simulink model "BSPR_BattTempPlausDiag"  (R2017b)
settings: Solver=FixedStepDiscrete  StartTime=0.0  StopTime=10.0  FixedStep=0.02  RelTol=1e-3  EnableMultiTasking=on
undefined symbols (not defined in the file): bin2dec, BSPR_cntBattTCnstErrDet_C, BSPR_cntBattTCnstErrHeal_C, BSPR_cntBattTHopErrDet_C, BSPR_cntBattTHopErrHeal_C, BSPR_cntBattTPlausDiag_CW, BSPR_cntCellTPlausDiag_CW, BSPR_cofBattTLowPassK_C, BSPR_tBattTCnstFaultThres_C, BSPR_tBattTempCnstHi_C, BSPR_tBattTempCnstLo_C, BSPR_tBattTempCnstThres_C, BSPR_tBattTempEnvtDiff_C, BSPR_tBattTHopFaultThres_C, BSPR_tBusbarTCnstFaultThres_C, BSPR_tBusbarTCnstHealThres_C, BSPR_tCellTCnstFaultThres_C, BSPR_tCellTCnstHealThres_C, BSPR_tiBattTCnstErrDet_C, BSPR_tiBattTCnstErrHeal_C
libraries: simulink x12
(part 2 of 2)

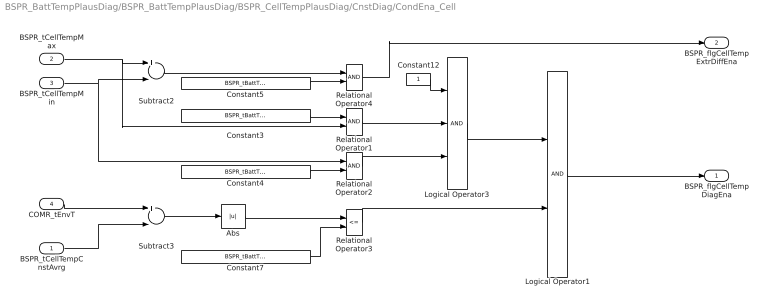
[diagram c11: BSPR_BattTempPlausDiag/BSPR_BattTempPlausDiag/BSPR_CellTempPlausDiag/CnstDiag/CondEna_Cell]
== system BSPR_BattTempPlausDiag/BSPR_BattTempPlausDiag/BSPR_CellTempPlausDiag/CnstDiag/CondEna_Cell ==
  BSPR_tCellTempCnstAvrg : Inport
  BSPR_tCellTempMax : Inport  Port=2
  BSPR_tCellTempMin : Inport  Port=3
  COMR_tEnvT : Inport  Port=4
  Abs : Abs
  Constant12 : Constant  OutDataTypeStr=boolean
  Constant3 : Constant  Value=BSPR_tBattTempCnstHi_C
  Constant4 : Constant  Value=BSPR_tBattTempCnstLo_C
  Constant5 : Constant  Value=BSPR_tBattTempCnstThres_C
  Constant7 : Constant  Value=BSPR_tBattTempEnvtDiff_C
  Logical Operator1 : Logic  AllPortsSameDT=off  OutDataTypeStr=boolean
  Logical Operator3 : Logic  Inputs=3  AllPortsSameDT=off  OutDataTypeStr=boolean
  Relational Operator1 : RelationalOperator  OutDataTypeStr=boolean  RndMeth=Simplest
  Relational Operator2 : RelationalOperator  OutDataTypeStr=boolean  RndMeth=Simplest
  Relational Operator3 : RelationalOperator  Operator=<=  OutDataTypeStr=boolean  RndMeth=Simplest
  Relational Operator4 : RelationalOperator  OutDataTypeStr=boolean  RndMeth=Simplest
  Subtract2 : Sum  Inputs=+-  OutDataTypeStr=uint8
  Subtract3 : Sum  Inputs=+-  OutDataTypeStr=single
  BSPR_flgCellTempDiagEna : Outport
  BSPR_flgCellTempExtrDiffEna : Outport  Port=2
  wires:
  Relational Operator4/1 -> BSPR_flgCellTempExtrDiffEna/1
  Relational Operator1/1 -> Logical Operator3/2
  Abs/1 -> Relational Operator3/1
  Logical Operator1/1 -> BSPR_flgCellTempDiagEna/1
  Relational Operator3/1 -> Logical Operator1/2
  Logical Operator3/1 -> Logical Operator1/1
  Constant7/1 -> Relational Operator3/2
  Subtract3/1 -> Abs/1
  BSPR_tCellTempCnstAvrg/1 -> Subtract3/2
  COMR_tEnvT/1 -> Subtract3/1
  Relational Operator2/1 -> Logical Operator3/3
  Constant4/1 -> Relational Operator2/2
  Constant3/1 -> Relational Operator1/1
  Subtract2/1 -> Relational Operator4/1
  Constant5/1 -> Relational Operator4/2
  BSPR_tCellTempMin/1 -> Subtract2/2, Relational Operator2/1
  BSPR_tCellTempMax/1 -> Subtract2/1, Relational Operator1/2
  Constant12/1 -> Logical Operator3/1

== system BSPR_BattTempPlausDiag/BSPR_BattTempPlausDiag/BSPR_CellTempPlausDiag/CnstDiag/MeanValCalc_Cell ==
  BSPR_cntCellTSnsrNum : Inport
  BSPR_tCellTemp_A : Inport  Port=2
  BSPR_tCellTempCnstAvrg : Inport  Port=3
  MeanValCalc_Cell : Stateflow chart  TreatAsAtomicUnit=on
  BSPR_tAvrgCellTempFlt : Outport
  BSPR_tSumCellTempVari : Outport  Port=2
  BSPR_tSumCellTempFlt : Outport  Port=3
  BSPR_tCellTempVari_A : Outport  Port=4
  BSPR_tAvrgCellTempVari : Outport  Port=5
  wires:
  BSPR_tCellTempCnstAvrg/1 -> MeanValCalc_Cell/2(BSPR_tBattTempCnstAvrg)
  BSPR_tCellTemp_A/1 -> MeanValCalc_Cell/1(BSPR_tBattTemp_A)
  MeanValCalc_Cell/4(BSPR_tBattTempVari_A) -> BSPR_tCellTempVari_A/1
  MeanValCalc_Cell/1(BSPR_tAvrgBattTempFlt) -> BSPR_tAvrgCellTempFlt/1
  MeanValCalc_Cell/2(BSPR_tSumBattTempVari) -> BSPR_tSumCellTempVari/1
  MeanValCalc_Cell/5(BSPR_tAvrgBattTempVari) -> BSPR_tAvrgCellTempVari/1
  MeanValCalc_Cell/3(BSPR_tSumBattTempFlt) -> BSPR_tSumCellTempFlt/1
  BSPR_cntCellTSnsrNum/1 -> MeanValCalc_Cell/3(BSPR_cntBattTSnsrNum)

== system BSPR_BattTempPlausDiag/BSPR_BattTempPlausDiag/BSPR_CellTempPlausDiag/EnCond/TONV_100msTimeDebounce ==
  note: Turn On Delay Time Deboune
  u : Inport
  T : Inport  Port=2
  Add : Sum
  Constant1 : Constant  Value=0  OutDataTypeStr=single
  Constant2 : Constant  OutDataTypeStr=uint8
  Constant3 : Constant  Value=0  OutDataTypeStr=uint8
  Constant4 : Constant  Value=0.1  OutDataTypeStr=single
  Delay : Delay  DelayLength=1  InitialCondition=0
  MinMax : MinMax  Inputs=2
  Product : Product  OutMin=[0]  OutMax=[65535]  OutDataTypeStr=single
  Relational Operator : RelationalOperator  Operator=>  OutDataTypeStr=boolean  RndMeth=Simplest
  Switch : Switch  Criteria=u2 ~= 0
  Switch1 : Switch  Criteria=u2 ~= 0
  y : Outport
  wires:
  MinMax/1 -> Add/2
  T/1 -> Relational Operator/2, MinMax/1
  Relational Operator/1 -> y/1
  Delay/1 -> MinMax/2
  Switch/1 -> Add/1
  Product/1 -> Delay/1, Relational Operator/1
  Add/1 -> Product/2
  Constant1/1 -> Switch/3
  Constant4/1 -> Switch/1
  u/1 -> Switch/2, Switch1/2
  Constant2/1 -> Switch1/1
  Constant3/1 -> Switch1/3
  Switch1/1 -> Product/1

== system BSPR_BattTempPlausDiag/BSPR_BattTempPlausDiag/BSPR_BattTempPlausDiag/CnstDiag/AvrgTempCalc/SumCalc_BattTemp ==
  BSPR_tBattTemp_A : Inport
  BSPR_cntBattTSnsrNum : Inport  Port=2
  SumCalc_BattTemp : Stateflow chart  TreatAsAtomicUnit=on
  BSPR_tSumBattTemp : Outport
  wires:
  BSPR_cntBattTSnsrNum/1 -> SumCalc_BattTemp/2(BSPR_cntBattTSnsrNum)
  BSPR_tBattTemp_A/1 -> SumCalc_BattTemp/1(BSPR_tBattTemp_A)
  SumCalc_BattTemp/1(BSPR_uSumBattTemp) -> BSPR_tSumBattTemp/1

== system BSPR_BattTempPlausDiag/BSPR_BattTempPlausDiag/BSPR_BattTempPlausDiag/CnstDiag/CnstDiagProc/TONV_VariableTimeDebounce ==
  note: Turn On Delay Time Deboune
  u : Inport
  T : Inport  Port=2
  dT : Inport  Port=3
  Add : Sum
  Constant1 : Constant  Value=0  OutDataTypeStr=single
  Constant2 : Constant  OutDataTypeStr=uint8
  Constant3 : Constant  Value=0  OutDataTypeStr=uint8
  Delay : Delay  DelayLength=1  InitialCondition=0
  MinMax : MinMax  Inputs=2
  Product : Product  OutMin=[0]  OutMax=[65535]  OutDataTypeStr=single
  Relational Operator : RelationalOperator  Operator=>  OutDataTypeStr=boolean  RndMeth=Simplest
  Switch : Switch  Criteria=u2 ~= 0
  Switch1 : Switch  Criteria=u2 ~= 0
  y : Outport
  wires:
  Switch1/1 -> Product/1
  Constant3/1 -> Switch1/3
  Constant2/1 -> Switch1/1
  u/1 -> Switch1/2, Switch/2
  dT/1 -> Switch/1
  Constant1/1 -> Switch/3
  Add/1 -> Product/2
  Product/1 -> Relational Operator/1, Delay/1
  Switch/1 -> Add/1
  Delay/1 -> MinMax/2
  Relational Operator/1 -> y/1
  T/1 -> MinMax/1, Relational Operator/2
  MinMax/1 -> Add/2

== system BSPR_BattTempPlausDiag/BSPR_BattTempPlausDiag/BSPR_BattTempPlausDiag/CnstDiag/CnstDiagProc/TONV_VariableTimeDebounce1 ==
  note: Turn On Delay Time Deboune
  u : Inport
  T : Inport  Port=2
  dT : Inport  Port=3
  Add : Sum
  Constant1 : Constant  Value=0  OutDataTypeStr=single
  Constant2 : Constant  OutDataTypeStr=uint8
  Constant3 : Constant  Value=0  OutDataTypeStr=uint8
  Delay : Delay  DelayLength=1  InitialCondition=0
  MinMax : MinMax  Inputs=2
  Product : Product  OutMin=[0]  OutMax=[65535]  OutDataTypeStr=single
  Relational Operator : RelationalOperator  Operator=>  OutDataTypeStr=boolean  RndMeth=Simplest
  Switch : Switch  Criteria=u2 ~= 0
  Switch1 : Switch  Criteria=u2 ~= 0
  y : Outport
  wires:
  MinMax/1 -> Add/2
  T/1 -> Relational Operator/2, MinMax/1
  Relational Operator/1 -> y/1
  Delay/1 -> MinMax/2
  Switch/1 -> Add/1
  Product/1 -> Delay/1, Relational Operator/1
  Add/1 -> Product/2
  Constant1/1 -> Switch/3
  dT/1 -> Switch/1
  u/1 -> Switch/2, Switch1/2
  Constant2/1 -> Switch1/1
  Constant3/1 -> Switch1/3
  Switch1/1 -> Product/1

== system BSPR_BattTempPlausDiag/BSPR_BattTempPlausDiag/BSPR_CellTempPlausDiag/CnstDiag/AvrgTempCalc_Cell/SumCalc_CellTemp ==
  BSPR_tCellTemp_A : Inport
  BSPR_cntCellTSnsrNum : Inport  Port=2
  SumCalc_CellTemp : Stateflow chart  TreatAsAtomicUnit=on
  BSPR_tSumCellTemp : Outport
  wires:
  SumCalc_CellTemp/1(BSPR_uSumBattTemp) -> BSPR_tSumCellTemp/1
  BSPR_tCellTemp_A/1 -> SumCalc_CellTemp/1(BSPR_tBattTemp_A)
  BSPR_cntCellTSnsrNum/1 -> SumCalc_CellTemp/2(BSPR_cntBattTSnsrNum)

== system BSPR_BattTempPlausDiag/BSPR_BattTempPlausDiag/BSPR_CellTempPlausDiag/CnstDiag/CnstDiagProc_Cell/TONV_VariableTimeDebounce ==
  note: Turn On Delay Time Deboune
  u : Inport
  T : Inport  Port=2
  dT : Inport  Port=3
  Add : Sum
  Constant1 : Constant  Value=0  OutDataTypeStr=single
  Constant2 : Constant  OutDataTypeStr=uint8
  Constant3 : Constant  Value=0  OutDataTypeStr=uint8
  Delay : Delay  DelayLength=1  InitialCondition=0
  MinMax : MinMax  Inputs=2
  Product : Product  OutMin=[0]  OutMax=[65535]  OutDataTypeStr=single
  Relational Operator : RelationalOperator  Operator=>  OutDataTypeStr=boolean  RndMeth=Simplest
  Switch : Switch  Criteria=u2 ~= 0
  Switch1 : Switch  Criteria=u2 ~= 0
  y : Outport
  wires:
  Switch1/1 -> Product/1
  Constant3/1 -> Switch1/3
  Constant2/1 -> Switch1/1
  u/1 -> Switch1/2, Switch/2
  dT/1 -> Switch/1
  Constant1/1 -> Switch/3
  Add/1 -> Product/2
  Product/1 -> Relational Operator/1, Delay/1
  Switch/1 -> Add/1
  Delay/1 -> MinMax/2
  Relational Operator/1 -> y/1
  T/1 -> MinMax/1, Relational Operator/2
  MinMax/1 -> Add/2

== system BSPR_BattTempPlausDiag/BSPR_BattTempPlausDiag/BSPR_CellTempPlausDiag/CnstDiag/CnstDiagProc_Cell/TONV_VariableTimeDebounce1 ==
  note: Turn On Delay Time Deboune
  u : Inport
  T : Inport  Port=2
  dT : Inport  Port=3
  Add : Sum
  Constant1 : Constant  Value=0  OutDataTypeStr=single
  Constant2 : Constant  OutDataTypeStr=uint8
  Constant3 : Constant  Value=0  OutDataTypeStr=uint8
  Delay : Delay  DelayLength=1  InitialCondition=0
  MinMax : MinMax  Inputs=2
  Product : Product  OutMin=[0]  OutMax=[65535]  OutDataTypeStr=single
  Relational Operator : RelationalOperator  Operator=>  OutDataTypeStr=boolean  RndMeth=Simplest
  Switch : Switch  Criteria=u2 ~= 0
  Switch1 : Switch  Criteria=u2 ~= 0
  y : Outport
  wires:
  MinMax/1 -> Add/2
  T/1 -> Relational Operator/2, MinMax/1
  Relational Operator/1 -> y/1
  Delay/1 -> MinMax/2
  Switch/1 -> Add/1
  Product/1 -> Delay/1, Relational Operator/1
  Add/1 -> Product/2
  Constant1/1 -> Switch/3
  dT/1 -> Switch/1
  u/1 -> Switch/2, Switch1/2
  Constant2/1 -> Switch1/1
  Constant3/1 -> Switch1/3
  Switch1/1 -> Product/1

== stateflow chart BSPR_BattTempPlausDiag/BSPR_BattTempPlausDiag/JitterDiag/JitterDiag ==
  state Ini_stt
    (default) -> (junction 142) : % ini
    (junction 138) -> (junction 143) : [i<BSPR_cntBattTSnsrNum]
    (junction 142) -> (junction 138) : {i=0;}
    (junction 143) -> (junction 139) : {BSPR_tBattTempDiag_A[i]=BSPR_tBattTemp_A[i]; BSPR_tBattTHopDiff_A[i]=0;}
    (junction 139) -> (junction 138) : {i = i + 1;}
    (junction 138) -> (junction 136)
  state DiagUCellProc_stt
    (default) -> (junction 10) : /*Compare */
    (junction 23) -> (junction 120) : [abs(BSPR_tBattTHopDiff_A[i])>=BSPR_tBattTHopFaultThres_C]
    (junction 9) -> (junction 23) : {[BSPR_tBattTempDiag_A[i],BSPR_tBattTHopDiff_A[i]]=LowPassK(BSPR_tBattTemp_A[i],BSPR_tBattTempDiag_A[i],BSPR_cofBattTLowPassK_C);}
    (junction 11) -> (junction 9) : [i<BSPR_cntBattTSnsrNum]
    (junction 10) -> (junction 11) : {i=0;}
    (junction 23) -> (junction 25) : {BSPR_bBattTHopErrStt_A[i]=0;}
    (junction 120) -> (junction 122) : {BSPR_bBattTHopErrStt_A[i]=1;}
    (junction 12) -> (junction 11) : {i = i + 1;}
    (junction 11) -> (junction 13) : /*Debounce*/
    (junction 25) -> (junction 12)
    (junction 122) -> (junction 25)
    (junction 48) -> (junction 41) : [BSPR_bBattTHopErrStt_A[i]==1]
    (junction 13) -> (junction 51) : {i=0;}
    (junction 51) -> (junction 48) : [i<BSPR_cntBattTSnsrNum]
    (junction 48) -> (junction 49) : {BSPR_cntBattTHopErrHeal_A[i]=BSPR_cntBattTHopErrHeal_A[i]+1; BSPR_cntBattTHopErrDet_A[i]=0;}
    (junction 41) -> (junction 42) : {BSPR_cntBattTHopErrDet_A[i]=BSPR_cntBattTHopErrDet_A[i]+1; BSPR_cntBattTHopErrHeal_A[i]=0;}
    (junction 49) -> (junction 51) : {i = i + 1;}
    (junction 51) -> (junction 86) : /*Output error result*/
    (junction 42) -> (junction 49)
    (junction 86) -> (junction 64) : {i=0;}
    (junction 55) -> (junction 56) : [BSPR_cntBattTHopErrDet_A[i] > BSPR_cntBattTHopErrDet_C]
    (junction 64) -> (junction 55) : [i<BSPR_cntBattTSnsrNum]
    (junction 55) -> (junction 58) : {BSPR_bBattTHopErrDet_A[i]=0;}
    (junction 56) -> (junction 57) : {BSPR_bBattTHopErrDet_A[i]=1; BSPR_cntBattTHopErrDet_A[i] = BSPR_cntBattTHopErrDet_C;}
    (junction 58) -> (junction 64) : {i = i + 1;}
    (junction 64) -> (junction 84) : /*Output ok result*/
    (junction 57) -> (junction 58)
    (junction 84) -> (junction 69) : {i=0;}
    (junction 67) -> (junction 73) : [BSPR_cntBattTHopErrHeal_A[i] > BSPR_cntBattTHopErrHeal_C]
    (junction 69) -> (junction 67) : [i<BSPR_cntBattTSnsrNum]
    (junction 67) -> (junction 70) : {BSPR_bBattTHopErrHeal_A[i]=0;}
    (junction 73) -> (junction 74) : {BSPR_bBattTHopErrHeal_A[i]=1; BSPR_cntBattTHopErrHeal_A[i] = BSPR_cntBattTHopErrHeal_C;}
    (junction 70) -> (junction 69) : {i = i + 1;}
    (junction 69) -> (junction 78)
    (junction 74) -> (junction 70)
  state DiagDisable_stt
    (default) -> (junction 173) : {i=0;}
    (junction 173) -> (junction 174) : [i<BSPR_cntBattTSnsrNum]
    (junction 174) -> (junction 171) : {BSPR_bBattTHopErrHeal_A[i]=1; BSPR_bBattTHopErrDet_A[i]=0; BSPR_bBattTHopErrStt_A[i]=0; BSPR_cntBattTHopErrHeal_A[i]=0; BSPR_cntBattTHopErrDet_A[i]=0;}
    (junction 171) -> (junction 173) : {i = i + 1;}
    (junction 173) -> (junction 198)
  state [Temp_Out,Temp_Diff]   =LowPassK(u,u_old,k) [function]
    (default) -> (junction 105)
    (junction 105) -> (junction 116) : {Temp_Diff=u-u_old; Temp_Out=u_old+Temp_Diff*k; Temp_Diff=u-Temp_Out;}
    (junction 116) -> (junction 118)
  (default) -> Ini_stt
  Ini_stt -> DiagUCellProc_stt : [BSPR_bBattTHopDiagSwt]
  Ini_stt -> DiagDisable_stt : [~BSPR_bBattTHopDiagSwt]
  DiagDisable_stt -> DiagUCellProc_stt : [BSPR_bBattTHopDiagSwt]
  DiagUCellProc_stt -> DiagDisable_stt : [~BSPR_bBattTHopDiagSwt]
  (junction 93) -> DiagUCellProc_stt
  (junction 91) -> (junction 93)
  DiagUCellProc_stt -> (junction 89)
  (junction 89) -> (junction 91)
  data: u function_input double; u_old function_input double; k function_input double; Temp_Out function_output double; Temp_Diff function_output double; BSPR_tBattTempDiag_A output; BSPR_tBattTHopDiff_A output; BSPR_bBattTHopErrStt_A output; BSPR_tBattTemp_A input; BSPR_cntBattTSnsrNum input; BSPR_cofBattTLowPassK_C input; BSPR_bBattTHopErrDet_A output; BSPR_bBattTHopErrHeal_A output; i local uint8; BSPR_tBattTHopFaultThres_C input; BSPR_cntBattTHopErrDet_C input; BSPR_cntBattTHopErrHeal_C input; BSPR_cntBattTHopErrDet_A output uint16; BSPR_cntBattTHopErrHeal_A output uint16; BSPR_bBattTHopDiagSwt input

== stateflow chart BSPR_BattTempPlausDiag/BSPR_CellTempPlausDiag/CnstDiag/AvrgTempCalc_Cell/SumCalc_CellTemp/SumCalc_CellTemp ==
  state SumBattTemp_Stt
    (default) -> (junction 10) : % SumBattTemp
    (junction 10) -> (junction 11) : {i=0;BSPR_uSumBattTemp=0;}
    (junction 11) -> (junction 9) : [i<BSPR_cntBattTSnsrNum]
    (junction 9) -> (junction 12) : {BSPR_uSumBattTemp=BSPR_uSumBattTemp+BSPR_tBattTemp_A[i];}
    (junction 12) -> (junction 11) : {i = i + 1;}
    (junction 11) -> (junction 13)
  (default) -> SumBattTemp_Stt
  (junction 25) -> SumBattTemp_Stt
  (junction 23) -> (junction 25)
  SumBattTemp_Stt -> (junction 20)
  (junction 20) -> (junction 23)
  data: BSPR_tBattTemp_A input; BSPR_uSumBattTemp output; BSPR_cntBattTSnsrNum input; i local uint8

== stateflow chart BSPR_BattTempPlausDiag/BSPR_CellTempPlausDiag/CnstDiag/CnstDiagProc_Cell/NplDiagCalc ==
  state CnstDiag_stt
    (default) -> (junction 96) : /*Condition */
    (junction 98) -> (junction 121) : [~BSPR_flgBattTempExtrDiffEna]
    (junction 96) -> (junction 98)
    (junction 121) -> (junction 126) : {i=0;}
    (junction 98) -> (junction 100) : [BSPR_flgBattTempExtrDiffEna]
    (junction 96) -> (junction 103) : [BSPR_flgBattTempDiagEna]
    (junction 103) -> (junction 10) : /*Compare */
    (junction 126) -> (junction 131) : [i<BSPR_cntBattTSnsrNum]
    (junction 9) -> (junction 23) : [(abs(BSPR_tBattTemp_A[i]-BSPR_tAvrgBattTempFlt)>=BSPR_tBattTCnstFaultThres_C)]
    (junction 11) -> (junction 9) : [i<BSPR_cntBattTSnsrNum]
    (junction 10) -> (junction 11) : {i=0;}
    (junction 131) -> (junction 132) : {BSPR_bBattTCnstErrHeal_A[i]=1; BSPR_bBattTCnstErrDet_A[i]=0; BSPR_bBattTCnstErrStt_A[i]=0; BSPR_cntBattTCnstErrHeal_A[i]=0; BSPR_cntBattTCnstErrDet_A[i]=0;}
    (junction 9) -> (junction 12) : {BSPR_bBattTCnstErrStt_A[i]=0;}
    (junction 23) -> (junction 25) : {BSPR_bBattTCnstErrStt_A[i]=1;}
    (junction 12) -> (junction 11) : {i = i + 1;}
    (junction 132) -> (junction 126) : {i = i + 1;}
    (junction 126) -> (junction 123)
    (junction 11) -> (junction 13) : /*Debounce*/
    (junction 25) -> (junction 12)
    (junction 48) -> (junction 41) : [BSPR_bBattTCnstErrStt_A[i]==1]
    (junction 13) -> (junction 51) : {i=0;}
    (junction 51) -> (junction 48) : [i<BSPR_cntBattTSnsrNum]
    (junction 48) -> (junction 49) : {BSPR_cntBattTCnstErrHeal_A[i]=BSPR_cntBattTCnstErrHeal_A[i]+1; BSPR_cntBattTCnstErrDet_A[i]=0;}
    (junction 41) -> (junction 42) : {BSPR_cntBattTCnstErrDet_A[i]=BSPR_cntBattTCnstErrDet_A[i]+1; BSPR_cntBattTCnstErrHeal_A[i]=0;}
    (junction 49) -> (junction 51) : {i = i + 1;}
    (junction 51) -> (junction 86) : /*Output error result*/
    (junction 42) -> (junction 49)
    (junction 86) -> (junction 64) : {i=0;}
    (junction 55) -> (junction 56) : [BSPR_cntBattTCnstErrDet_A[i] > BSPR_cntBattTCnstErrDet_C]
    (junction 64) -> (junction 55) : [i<BSPR_cntBattTSnsrNum]
    (junction 55) -> (junction 58) : {BSPR_bBattTCnstErrDet_A[i]=0;}
    (junction 56) -> (junction 57) : {BSPR_bBattTCnstErrDet_A[i]=1; BSPR_cntBattTCnstErrDet_A[i] = BSPR_cntBattTCnstErrDet_C;}
    (junction 58) -> (junction 64) : {i = i + 1;}
    (junction 64) -> (junction 84) : /*Output ok result*/
    (junction 57) -> (junction 58)
    (junction 84) -> (junction 69) : {i=0;}
    (junction 67) -> (junction 73) : [BSPR_cntBattTCnstErrHeal_A[i] > BSPR_cntBattTCnstErrHeal_C]
    (junction 69) -> (junction 67) : [i<BSPR_cntBattTSnsrNum]
    (junction 67) -> (junction 70) : {BSPR_bBattTCnstErrHeal_A[i]=0;}
    (junction 73) -> (junction 74) : {BSPR_bBattTCnstErrHeal_A[i]=1; BSPR_cntBattTCnstErrHeal_A[i] = BSPR_cntBattTCnstErrHeal_C;}
    (junction 70) -> (junction 69) : {i = i + 1;}
    (junction 69) -> (junction 78)
    (junction 74) -> (junction 70)
    (junction 123) -> (junction 100)
    (junction 100) -> (junction 78)
    (junction 78) -> (junction 105)
  state DiagDisable_stt
    (default) -> (junction 115) : {i=0;}
    (junction 115) -> (junction 110) : [i<BSPR_cntBattTSnsrNum]
    (junction 110) -> (junction 108) : {BSPR_bBattTCnstErrHeal_A[i]=1; BSPR_bBattTCnstErrDet_A[i]=0; BSPR_bBattTCnstErrStt_A[i]=0; BSPR_cntBattTCnstErrHeal_A[i]=0; BSPR_cntBattTCnstErrDet_A[i]=0;}
    (junction 108) -> (junction 115) : {i = i + 1;}
    (junction 115) -> (junction 113)
  (default) -> CnstDiag_stt
  CnstDiag_stt -> DiagDisable_stt : [~BSPR_bBattTCnstDiagSwt]
  DiagDisable_stt -> CnstDiag_stt : [BSPR_bBattTCnstDiagSwt]
  (junction 93) -> CnstDiag_stt
  (junction 91) -> (junction 93)
  CnstDiag_stt -> (junction 89) : [BSPR_bBattTCnstDiagSwt]
  (junction 89) -> (junction 91)
  data: BSPR_tBattTemp_A input; BSPR_tAvrgBattTempFlt input; BSPR_bBattTCnstErrDet_A output; BSPR_flgBattTempDiagEna input; BSPR_flgBattTempExtrDiffEna input; BSPR_cntBattTSnsrNum input; i local uint8; BSPR_tBattTCnstFaultThres_C input; BSPR_bBattTCnstErrHeal_A output; BSPR_cntBattTCnstErrDet_C input; BSPR_cntBattTCnstErrHeal_C input; BSPR_bBattTCnstErrStt_A output; BSPR_cntBattTCnstErrDet_A output uint16; BSPR_cntBattTCnstErrHeal_A output uint16; BSPR_bBattTCnstDiagSwt input

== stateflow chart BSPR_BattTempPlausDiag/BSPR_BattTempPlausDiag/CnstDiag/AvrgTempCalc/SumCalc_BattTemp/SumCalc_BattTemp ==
  state SumBattTemp_Stt
    (default) -> (junction 10) : % SumBattTemp
    (junction 10) -> (junction 11) : {i=0;BSPR_uSumBattTemp=0;}
    (junction 11) -> (junction 9) : [i<BSPR_cntBattTSnsrNum]
    (junction 9) -> (junction 12) : {BSPR_uSumBattTemp=BSPR_uSumBattTemp+BSPR_tBattTemp_A[i];}
    (junction 12) -> (junction 11) : {i = i + 1;}
    (junction 11) -> (junction 13)
  (default) -> SumBattTemp_Stt
  (junction 25) -> SumBattTemp_Stt
  (junction 23) -> (junction 25)
  SumBattTemp_Stt -> (junction 20)
  (junction 20) -> (junction 23)
  data: BSPR_tBattTemp_A input; BSPR_uSumBattTemp output; BSPR_cntBattTSnsrNum input; i local uint8

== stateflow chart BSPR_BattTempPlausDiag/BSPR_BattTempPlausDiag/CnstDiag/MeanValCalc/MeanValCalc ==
  state MeanVal_stt
    (default) -> (junction 70) : % Ini
    (junction 66) -> (junction 62) : [i<BSPR_cntBattTSnsrNum]
    (junction 70) -> (junction 66) : {i=0;}
    (junction 62) -> (junction 65) : {BSPR_tBattTempVari_A[i]=0;}
    (junction 65) -> (junction 66) : {i = i + 1;}
    (junction 66) -> (junction 10) : % SumVariance
    (junction 10) -> (junction 11) : {i=0;BSPR_tSumBattTempVari=0;}
    (junction 11) -> (junction 9) : [i<BSPR_cntBattTSnsrNum]
    (junction 9) -> (junction 12) : {BSPR_tBattTempDiffTmp=abs(BSPR_tBattTemp_A[i] - BSPR_tBattTempCnstAvrg); BSPR_tBattTempVari_A[i]=BSPR_tBattTempDiffTmp^2; BSPR_tSumBattTempVari=BSPR_tSumBattTempVari+BSPR_tBattTempVari_A[i];}
    (junction 12) -> (junction 11) : {i = i + 1;}
    (junction 11) -> (junction 13) : % AvrgCalc
    (junction 13) -> (junction 52) : {BSPR_tAvrgBattTempVari=BSPR_tSumBattTempVari/BSPR_cntBattTSnsrNum;}
    (junction 29) -> (junction 39) : [BSPR_tBattTempVari_A[i]>BSPR_tAvrgBattTempVari]
    (junction 34) -> (junction 29) : [i<BSPR_cntBattTSnsrNum]
    (junction 52) -> (junction 34) : {i=0; SumCnt=0; BSPR_tSumBattTempFlt=0; BSPR_tAvrgBattTempFlt=0;}
    (junction 29) -> (junction 32) : {BSPR_tSumBattTempFlt=BSPR_tBattTemp_A[i]+BSPR_tSumBattTempFlt; SumCnt=SumCnt+1;}
    (junction 39) -> (junction 37)
    (junction 32) -> (junction 34) : {i = i + 1;}
    (junction 34) -> (junction 35)
    (junction 37) -> (junction 32)
    (junction 35) -> (junction 72) : [SumCnt < 1]{BSPR_tAvrgBattTempFlt=BSPR_tSumBattTempFlt;}
    (junction 72) -> (junction 44)
    (junction 35) -> (junction 44) : {BSPR_tAvrgBattTempFlt=BSPR_tSumBattTempFlt/SumCnt;}
  (default) -> MeanVal_stt
  (junction 59) -> MeanVal_stt
  (junction 57) -> (junction 59)
  MeanVal_stt -> (junction 55)
  (junction 55) -> (junction 57)
  data: BSPR_tAvrgBattTempFlt output; BSPR_tBattTemp_A input; BSPR_tBattTempCnstAvrg input; BSPR_tSumBattTempVari output; BSPR_cntBattTSnsrNum input; i local uint8; BSPR_tSumBattTempFlt output; BSPR_tBattTempVari_A output; BSPR_tAvrgBattTempVari output; SumCnt local uint8; BSPR_tBattTempDiffTmp local single

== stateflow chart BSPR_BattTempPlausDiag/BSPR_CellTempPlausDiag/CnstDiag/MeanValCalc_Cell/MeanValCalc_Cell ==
  state MeanVal_stt
    (default) -> (junction 70) : % Ini
    (junction 66) -> (junction 62) : [i<BSPR_cntBattTSnsrNum]
    (junction 70) -> (junction 66) : {i=0;}
    (junction 62) -> (junction 65) : {BSPR_tBattTempVari_A[i]=0;}
    (junction 65) -> (junction 66) : {i = i + 1;}
    (junction 66) -> (junction 10) : % SumVariance
    (junction 10) -> (junction 11) : {i=0;BSPR_tSumBattTempVari=0;}
    (junction 11) -> (junction 9) : [i<BSPR_cntBattTSnsrNum]
    (junction 9) -> (junction 12) : {BSPR_tBattTempDiffTmp=abs(BSPR_tBattTemp_A[i] - BSPR_tBattTempCnstAvrg); BSPR_tBattTempVari_A[i]=BSPR_tBattTempDiffTmp^2; BSPR_tSumBattTempVari=BSPR_tSumBattTempVari+BSPR_tBattTempVari_A[i];}
    (junction 12) -> (junction 11) : {i = i + 1;}
    (junction 11) -> (junction 13) : % AvrgCalc
    (junction 13) -> (junction 52) : {BSPR_tAvrgBattTempVari=BSPR_tSumBattTempVari/BSPR_cntBattTSnsrNum;}
    (junction 29) -> (junction 39) : [BSPR_tBattTempVari_A[i]>BSPR_tAvrgBattTempVari]
    (junction 34) -> (junction 29) : [i<BSPR_cntBattTSnsrNum]
    (junction 52) -> (junction 34) : {i=0; SumCnt=0; BSPR_tSumBattTempFlt=0; BSPR_tAvrgBattTempFlt=0;}
    (junction 29) -> (junction 32) : {BSPR_tSumBattTempFlt=BSPR_tBattTemp_A[i]+BSPR_tSumBattTempFlt; SumCnt=SumCnt+1;}
    (junction 39) -> (junction 37)
    (junction 32) -> (junction 34) : {i = i + 1;}
    (junction 34) -> (junction 35)
    (junction 37) -> (junction 32)
    (junction 35) -> (junction 72) : [SumCnt < 1]{BSPR_tAvrgBattTempFlt=BSPR_tSumBattTempFlt;}
    (junction 72) -> (junction 44)
    (junction 35) -> (junction 44) : {BSPR_tAvrgBattTempFlt=BSPR_tSumBattTempFlt/SumCnt;}
  (default) -> MeanVal_stt
  (junction 59) -> MeanVal_stt
  (junction 57) -> (junction 59)
  MeanVal_stt -> (junction 55)
  (junction 55) -> (junction 57)
  data: BSPR_tAvrgBattTempFlt output; BSPR_tBattTemp_A input; BSPR_tBattTempCnstAvrg input; BSPR_tSumBattTempVari output; BSPR_cntBattTSnsrNum input; i local uint8; BSPR_tSumBattTempFlt output; BSPR_tBattTempVari_A output; BSPR_tAvrgBattTempVari output; SumCnt local uint8; BSPR_tBattTempDiffTmp local single

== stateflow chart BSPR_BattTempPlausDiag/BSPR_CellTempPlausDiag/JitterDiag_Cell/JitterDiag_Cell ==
  state Ini_stt
    (default) -> (junction 142) : % ini
    (junction 138) -> (junction 143) : [i<BSPR_cntBattTSnsrNum]
    (junction 142) -> (junction 138) : {i=0;}
    (junction 143) -> (junction 139) : {BSPR_tBattTempDiag_A[i]=BSPR_tBattTemp_A[i]; BSPR_tBattTHopDiff_A[i]=0;}
    (junction 139) -> (junction 138) : {i = i + 1;}
    (junction 138) -> (junction 136)
  state DiagUCellProc_stt
    (default) -> (junction 10) : /*Compare */
    (junction 23) -> (junction 120) : [abs(BSPR_tBattTHopDiff_A[i])>=BSPR_tBattTHopFaultThres_C]
    (junction 9) -> (junction 23) : {[BSPR_tBattTempDiag_A[i],BSPR_tBattTHopDiff_A[i]]=LowPassK(BSPR_tBattTemp_A[i],BSPR_tBattTempDiag_A[i],BSPR_cofBattTLowPassK_C);}
    (junction 11) -> (junction 9) : [i<BSPR_cntBattTSnsrNum]
    (junction 10) -> (junction 11) : {i=0;}
    (junction 23) -> (junction 25) : {BSPR_bBattTHopErrStt_A[i]=0;}
    (junction 120) -> (junction 122) : {BSPR_bBattTHopErrStt_A[i]=1;}
    (junction 12) -> (junction 11) : {i = i + 1;}
    (junction 11) -> (junction 13) : /*Debounce*/
    (junction 25) -> (junction 12)
    (junction 122) -> (junction 25)
    (junction 48) -> (junction 41) : [BSPR_bBattTHopErrStt_A[i]==1]
    (junction 13) -> (junction 51) : {i=0;}
    (junction 51) -> (junction 48) : [i<BSPR_cntBattTSnsrNum]
    (junction 48) -> (junction 49) : {BSPR_cntBattTHopErrHeal_A[i]=BSPR_cntBattTHopErrHeal_A[i]+1; BSPR_cntBattTHopErrDet_A[i]=0;}
    (junction 41) -> (junction 42) : {BSPR_cntBattTHopErrDet_A[i]=BSPR_cntBattTHopErrDet_A[i]+1; BSPR_cntBattTHopErrHeal_A[i]=0;}
    (junction 49) -> (junction 51) : {i = i + 1;}
    (junction 51) -> (junction 86) : /*Output error result*/
    (junction 42) -> (junction 49)
    (junction 86) -> (junction 64) : {i=0;}
    (junction 55) -> (junction 56) : [BSPR_cntBattTHopErrDet_A[i] > BSPR_cntBattTHopErrDet_C]
    (junction 64) -> (junction 55) : [i<BSPR_cntBattTSnsrNum]
    (junction 55) -> (junction 58) : {BSPR_bBattTHopErrDet_A[i]=0;}
    (junction 56) -> (junction 57) : {BSPR_bBattTHopErrDet_A[i]=1; BSPR_cntBattTHopErrDet_A[i] = BSPR_cntBattTHopErrDet_C;}
    (junction 58) -> (junction 64) : {i = i + 1;}
    (junction 64) -> (junction 84) : /*Output ok result*/
    (junction 57) -> (junction 58)
    (junction 84) -> (junction 69) : {i=0;}
    (junction 67) -> (junction 73) : [BSPR_cntBattTHopErrHeal_A[i] > BSPR_cntBattTHopErrHeal_C]
    (junction 69) -> (junction 67) : [i<BSPR_cntBattTSnsrNum]
    (junction 67) -> (junction 70) : {BSPR_bBattTHopErrHeal_A[i]=0;}
    (junction 73) -> (junction 74) : {BSPR_bBattTHopErrHeal_A[i]=1; BSPR_cntBattTHopErrHeal_A[i] = BSPR_cntBattTHopErrHeal_C;}
    (junction 70) -> (junction 69) : {i = i + 1;}
    (junction 69) -> (junction 78)
    (junction 74) -> (junction 70)
  state DiagDisable_stt
    (default) -> (junction 173) : {i=0;}
    (junction 173) -> (junction 174) : [i<BSPR_cntBattTSnsrNum]
    (junction 174) -> (junction 171) : {BSPR_bBattTHopErrHeal_A[i]=1; BSPR_bBattTHopErrDet_A[i]=0; BSPR_bBattTHopErrStt_A[i]=0; BSPR_cntBattTHopErrHeal_A[i]=0; BSPR_cntBattTHopErrDet_A[i]=0;}
    (junction 171) -> (junction 173) : {i = i + 1;}
    (junction 173) -> (junction 198)
  state [Temp_Out,Temp_Diff]   =LowPassK(u,u_old,k) [function]
    (default) -> (junction 105)
    (junction 105) -> (junction 116) : {Temp_Diff=u-u_old; Temp_Out=u_old+Temp_Diff*k; Temp_Diff=u-Temp_Out;}
    (junction 116) -> (junction 118)
  (default) -> Ini_stt
  Ini_stt -> DiagUCellProc_stt : [BSPR_bBattTHopDiagSwt]
  Ini_stt -> DiagDisable_stt : [~BSPR_bBattTHopDiagSwt]
  DiagDisable_stt -> DiagUCellProc_stt : [BSPR_bBattTHopDiagSwt]
  DiagUCellProc_stt -> DiagDisable_stt : [~BSPR_bBattTHopDiagSwt]
  (junction 93) -> DiagUCellProc_stt
  (junction 91) -> (junction 93)
  DiagUCellProc_stt -> (junction 89)
  (junction 89) -> (junction 91)
  data: u function_input double; u_old function_input double; k function_input double; Temp_Out function_output double; Temp_Diff function_output double; BSPR_tBattTempDiag_A output; BSPR_tBattTHopDiff_A output; BSPR_bBattTHopErrStt_A output; BSPR_tBattTemp_A input; BSPR_cntBattTSnsrNum input; BSPR_cofBattTLowPassK_C input; BSPR_bBattTHopErrDet_A output; BSPR_bBattTHopErrHeal_A output; i local uint8; BSPR_tBattTHopFaultThres_C input; BSPR_cntBattTHopErrDet_C input; BSPR_cntBattTHopErrHeal_C input; BSPR_cntBattTHopErrDet_A output uint16; BSPR_cntBattTHopErrHeal_A output uint16; BSPR_bBattTHopDiagSwt input

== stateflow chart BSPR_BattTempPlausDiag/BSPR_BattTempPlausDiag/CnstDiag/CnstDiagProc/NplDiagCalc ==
  state CnstDiag_stt
    (default) -> (junction 96) : /*Condition */
    (junction 98) -> (junction 121) : [~BSPR_flgBattTempExtrDiffEna]
    (junction 96) -> (junction 98)
    (junction 121) -> (junction 126) : {i=0;}
    (junction 98) -> (junction 100) : [BSPR_flgBattTempExtrDiffEna]
    (junction 96) -> (junction 103) : [BSPR_flgBattTempDiagEna]
    (junction 103) -> (junction 10) : /*Compare */
    (junction 126) -> (junction 131) : [i<BSPR_cntBattTSnsrNum]
    (junction 9) -> (junction 23) : [(abs(BSPR_tBattTemp_A[i]-BSPR_tAvrgBattTempFlt)>=BSPR_tBattTCnstFaultThres_C)]
    (junction 11) -> (junction 9) : [i<BSPR_cntBattTSnsrNum]
    (junction 10) -> (junction 11) : {i=0;}
    (junction 131) -> (junction 132) : {BSPR_bBattTCnstErrHeal_A[i]=1; BSPR_bBattTCnstErrDet_A[i]=0; BSPR_bBattTCnstErrStt_A[i]=0; BSPR_cntBattTCnstErrHeal_A[i]=0; BSPR_cntBattTCnstErrDet_A[i]=0;}
    (junction 9) -> (junction 12) : {BSPR_bBattTCnstErrStt_A[i]=0;}
    (junction 23) -> (junction 25) : {BSPR_bBattTCnstErrStt_A[i]=1;}
    (junction 12) -> (junction 11) : {i = i + 1;}
    (junction 132) -> (junction 126) : {i = i + 1;}
    (junction 126) -> (junction 123)
    (junction 11) -> (junction 13) : /*Debounce*/
    (junction 25) -> (junction 12)
    (junction 48) -> (junction 41) : [BSPR_bBattTCnstErrStt_A[i]==1]
    (junction 13) -> (junction 51) : {i=0;}
    (junction 51) -> (junction 48) : [i<BSPR_cntBattTSnsrNum]
    (junction 48) -> (junction 49) : {BSPR_cntBattTCnstErrHeal_A[i]=BSPR_cntBattTCnstErrHeal_A[i]+1; BSPR_cntBattTCnstErrDet_A[i]=0;}
    (junction 41) -> (junction 42) : {BSPR_cntBattTCnstErrDet_A[i]=BSPR_cntBattTCnstErrDet_A[i]+1; BSPR_cntBattTCnstErrHeal_A[i]=0;}
    (junction 49) -> (junction 51) : {i = i + 1;}
    (junction 51) -> (junction 86) : /*Output error result*/
    (junction 42) -> (junction 49)
    (junction 86) -> (junction 64) : {i=0;}
    (junction 55) -> (junction 56) : [BSPR_cntBattTCnstErrDet_A[i] > BSPR_cntBattTCnstErrDet_C]
    (junction 64) -> (junction 55) : [i<BSPR_cntBattTSnsrNum]
    (junction 55) -> (junction 58) : {BSPR_bBattTCnstErrDet_A[i]=0;}
    (junction 56) -> (junction 57) : {BSPR_bBattTCnstErrDet_A[i]=1; BSPR_cntBattTCnstErrDet_A[i] = BSPR_cntBattTCnstErrDet_C;}
    (junction 58) -> (junction 64) : {i = i + 1;}
    (junction 64) -> (junction 84) : /*Output ok result*/
    (junction 57) -> (junction 58)
    (junction 84) -> (junction 69) : {i=0;}
    (junction 67) -> (junction 73) : [BSPR_cntBattTCnstErrHeal_A[i] > BSPR_cntBattTCnstErrHeal_C]
    (junction 69) -> (junction 67) : [i<BSPR_cntBattTSnsrNum]
    (junction 67) -> (junction 70) : {BSPR_bBattTCnstErrHeal_A[i]=0;}
    (junction 73) -> (junction 74) : {BSPR_bBattTCnstErrHeal_A[i]=1; BSPR_cntBattTCnstErrHeal_A[i] = BSPR_cntBattTCnstErrHeal_C;}
    (junction 70) -> (junction 69) : {i = i + 1;}
    (junction 69) -> (junction 78)
    (junction 74) -> (junction 70)
    (junction 123) -> (junction 100)
    (junction 100) -> (junction 78)
    (junction 78) -> (junction 105)
  state DiagDisable_stt
    (default) -> (junction 115) : {i=0;}
    (junction 115) -> (junction 110) : [i<BSPR_cntBattTSnsrNum]
    (junction 110) -> (junction 108) : {BSPR_bBattTCnstErrHeal_A[i]=1; BSPR_bBattTCnstErrDet_A[i]=0; BSPR_bBattTCnstErrStt_A[i]=0; BSPR_cntBattTCnstErrHeal_A[i]=0; BSPR_cntBattTCnstErrDet_A[i]=0;}
    (junction 108) -> (junction 115) : {i = i + 1;}
    (junction 115) -> (junction 113)
  (default) -> CnstDiag_stt
  CnstDiag_stt -> DiagDisable_stt : [~BSPR_bBattTCnstDiagSwt]
  DiagDisable_stt -> CnstDiag_stt : [BSPR_bBattTCnstDiagSwt]
  (junction 93) -> CnstDiag_stt
  (junction 91) -> (junction 93)
  CnstDiag_stt -> (junction 89) : [BSPR_bBattTCnstDiagSwt]
  (junction 89) -> (junction 91)
  data: BSPR_tBattTemp_A input; BSPR_tAvrgBattTempFlt input; BSPR_bBattTCnstErrDet_A output; BSPR_flgBattTempDiagEna input; BSPR_flgBattTempExtrDiffEna input; BSPR_cntBattTSnsrNum input; i local uint8; BSPR_tBattTCnstFaultThres_C input; BSPR_bBattTCnstErrHeal_A output; BSPR_cntBattTCnstErrDet_C input; BSPR_cntBattTCnstErrHeal_C input; BSPR_bBattTCnstErrStt_A output; BSPR_cntBattTCnstErrDet_A output uint16; BSPR_cntBattTCnstErrHeal_A output uint16; BSPR_bBattTCnstDiagSwt input
